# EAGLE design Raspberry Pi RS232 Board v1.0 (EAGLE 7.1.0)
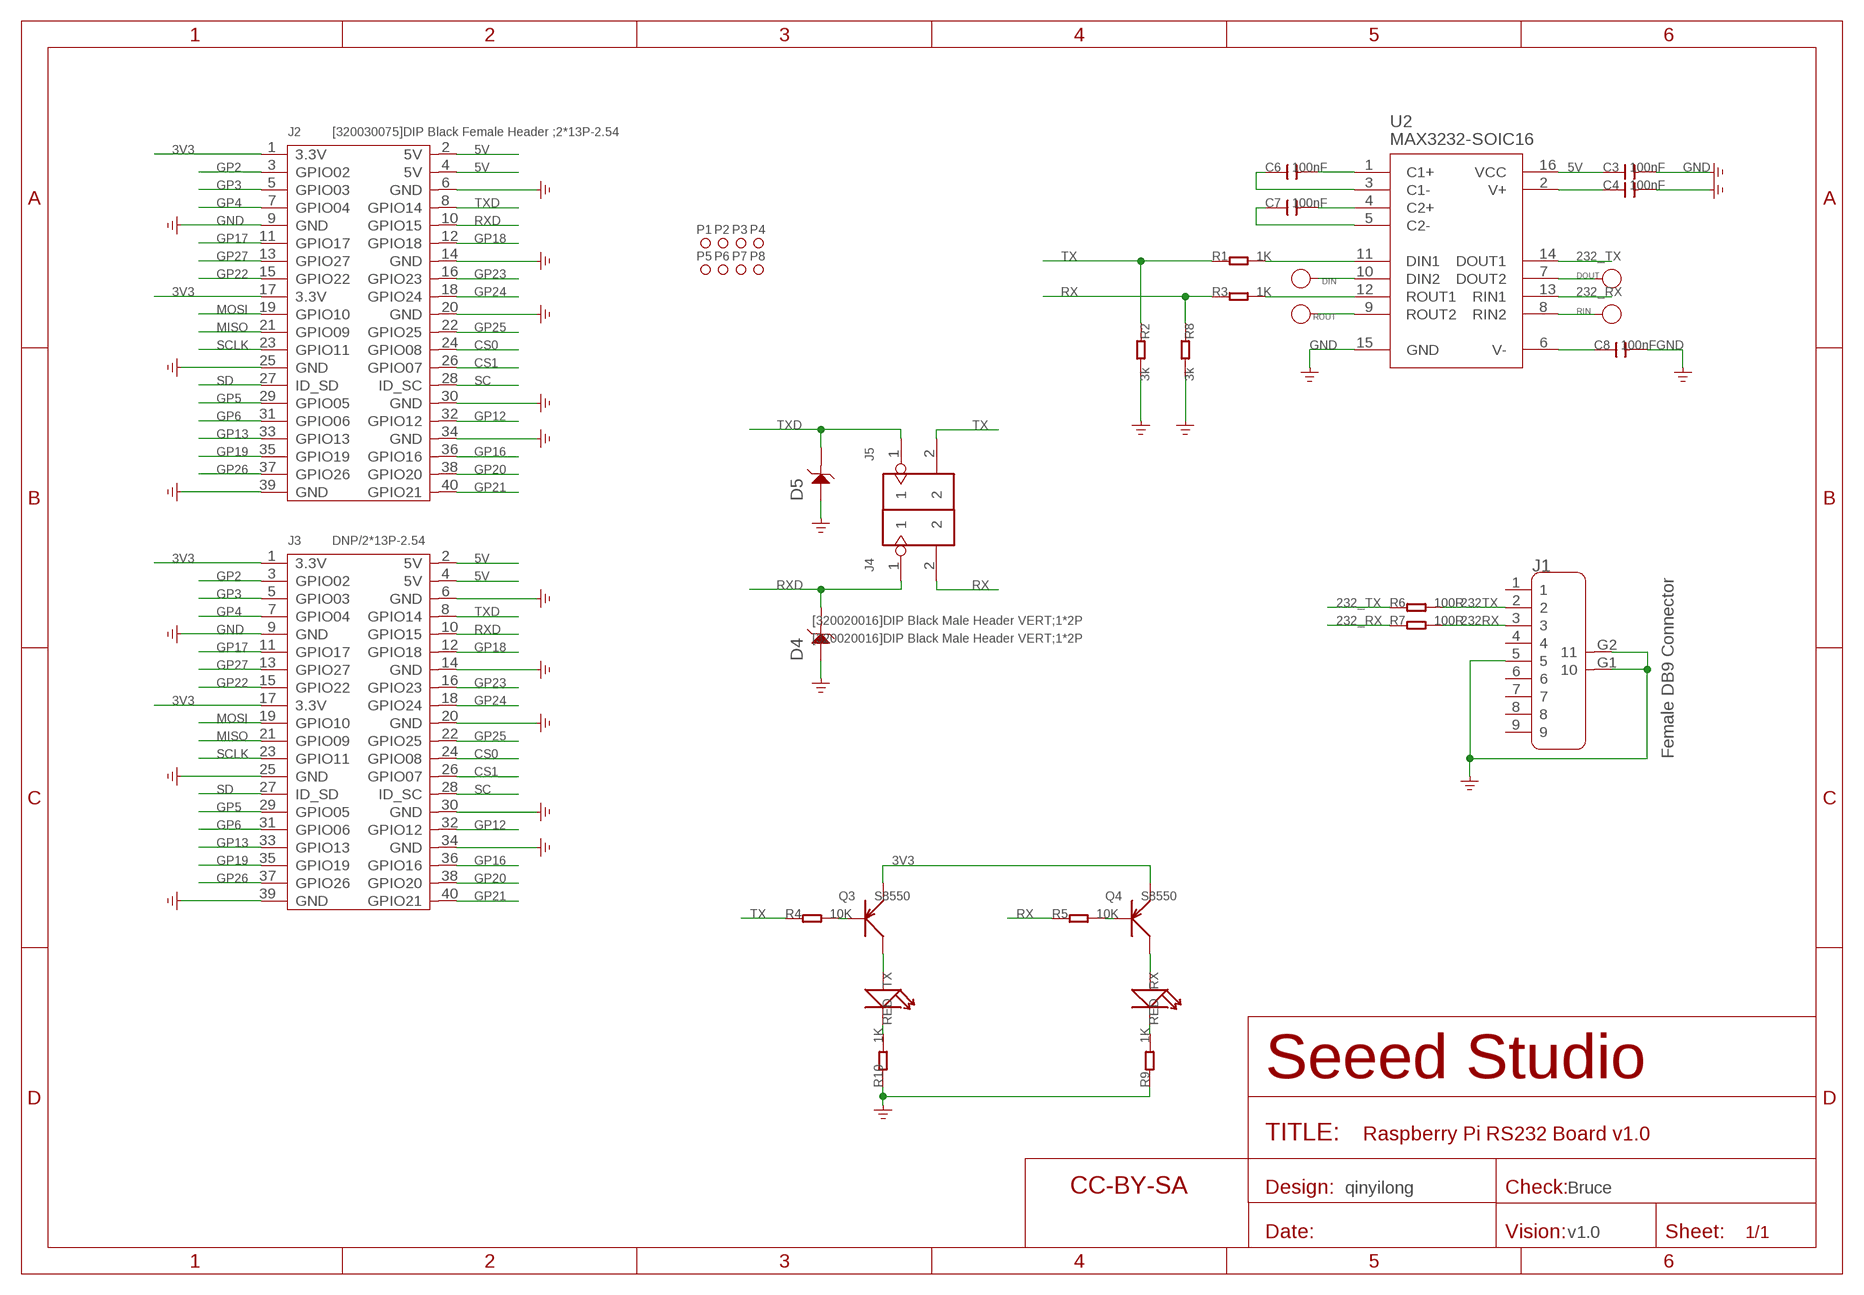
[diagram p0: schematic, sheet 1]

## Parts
C3  100nF  C-0603  [C0603]
C4  100nF  C-0603  [C0603]
C6  100nF  C-0603  [C0603]
C7  100nF  C-0603  [C0603]
C8  100nF  C-0603  [C0603]
D4  DNP  D-ESD-2P'CESD5V0D1'  [SOD123-2.7X1.6]
D5  DNP  D-ESD-2P'CESD5V0D1'  [SOD123-2.7X1.6]
DIN  DNP  PAD-TEST-POINT'4080'  [PAD_4080]
DOUT  DNP  PAD-TEST-POINT'4080'  [PAD_4080]
J1  Female DB9 Connector  DB9'FEMAL'  [DB9]
J2  [320030075]DIP Black Female Header ;2*13P-2.54  HEADER-2X20P  [2X20P-2.54-65/35MIL]
J3  DNP/2*13P-2.54  HEADER-2X20P  [2X20P-2.54-65/35MIL]
J4  [320020016]DIP Black Male Header VERT;1*2P  HEADER-2P-65/35MIL  [2P-2.54-65/35MIL]
J5  [320020016]DIP Black Male Header VERT;1*2P  HEADER-2P-65/35MIL  [2P-2.54-65/35MIL]
P1  PAD-MARK'ANNULAR'  [ROUND-MARK-1.0]
P2  PAD-MARK'ANNULAR'  [ROUND-MARK-1.0]
P3  PAD-MARK'ANNULAR'  [ROUND-MARK-1.0]
P4  PAD-MARK'ANNULAR'  [ROUND-MARK-1.0]
P5  PAD-MARK'ANNULAR'  [ROUND-MARK-1.0]
P6  PAD-MARK'ANNULAR'  [ROUND-MARK-1.0]
P7  PAD-MARK'ANNULAR'  [ROUND-MARK-1.0]
P8  PAD-MARK'ANNULAR'  [ROUND-MARK-1.0]
Q3  S8550  TRANSISTOR-PNP-SOT23  [SOT23]
Q4  S8550  TRANSISTOR-PNP-SOT23  [SOT23]
R1  1K  R-0603  [R0603]
R2  3k  R-0603  [R0603]
R3  1K  R-0603  [R0603]
R4  10K  R-0603  [R0603]
R5  10K  R-0603  [R0603]
R6  100R  R-0603  [R0603]
R7  100R  R-0603  [R0603]
R8  3k  R-0603  [R0603]
R9  1K  R-0603  [R0603]
R10  1K  R-0603  [R0603]
RIN  DNP  PAD-TEST-POINT'4080'  [PAD_4080]
ROUT  DNP  PAD-TEST-POINT'4080'  [PAD_4080]
RX  RED  LED'0603'  [LED-0603]
TX  RED  LED'0603'  [LED-0603]
U2  MAX3232-SOIC16  [SOIC16]
U$2  SEEEDSTUDIO-OPEN-SCH-FRAME  [SEEEDSTUDIO-PCB-FRAME]

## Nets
3V3: J2.1(3.3V) J2.17(3.3V) J3.1(3.3V) J3.17(3.3V) Q3.2(E) Q4.2(E)
5V: C3.1 J2.2(5V) J2.4(5V) J3.2(5V) J3.4(5V) U2.16(VCC)
232_RX: R7.1 U2.13(RIN1)
232_TX: R6.1 U2.14(DOUT1)
232RX: J1.3 R7.2
232TX: J1.2 R6.2
CS0: J2.24(GPIO08) J3.24(GPIO08)
CS1: J2.26(GPIO07) J3.26(GPIO07)
GND: C3.2 C4.2 C8.2 D4.1 D5.1 J1.5 J1.G1 J1.G2 J2.6(GND) J2.9(GND) J2.14(GND) J2.20(GND) J2.25(GND) J2.30(GND) J2.34(GND) J2.39(GND) J3.6(GND) J3.9(GND) J3.14(GND) J3.20(GND) J3.25(GND) J3.30(GND) J3.34(GND) J3.39(GND) R2.2 R8.2 R9.1 R10.1 U2.15(GND) ; supply symbol labelled GND_POWER
GP2: J2.3(GPIO02) J3.3(GPIO02)
GP3: J2.5(GPIO03) J3.5(GPIO03)
GP4: J2.7(GPIO04) J3.7(GPIO04)
GP5: J2.29(GPIO05) J3.29(GPIO05)
GP6: J2.31(GPIO06) J3.31(GPIO06)
GP12: J2.32(GPIO12) J3.32(GPIO12)
GP13: J2.33(GPIO13) J3.33(GPIO13)
GP16: J2.36(GPIO16) J3.36(GPIO16)
GP17: J2.11(GPIO17) J3.11(GPIO17)
GP18: J2.12(GPIO18) J3.12(GPIO18)
GP19: J2.35(GPIO19) J3.35(GPIO19)
GP20: J2.38(GPIO20) J3.38(GPIO20)
GP21: J2.40(GPIO21) J3.40(GPIO21)
GP22: J2.15(GPIO22) J3.15(GPIO22)
GP23: J2.16(GPIO23) J3.16(GPIO23)
GP24: J2.18(GPIO24) J3.18(GPIO24)
GP25: J2.22(GPIO25) J3.22(GPIO25)
GP26: J2.37(GPIO26) J3.37(GPIO26)
GP27: J2.13(GPIO27) J3.13(GPIO27)
MISO: J2.21(GPIO09) J3.21(GPIO09)
MOSI: J2.19(GPIO10) J3.19(GPIO10)
N$1: C6.2 U2.1(C1+)
N$3: C6.1 U2.3(C1-)
N$5: DIN.1(T) U2.10(DIN2)
N$6: ROUT.1(T) U2.9(ROUT2)
N$7: C7.2 U2.4(C2+)
N$8: C7.1 U2.5(C2-)
N$9: C8.1 U2.6(V-)
N$10: C4.1 U2.2(V+)
N$11: Q3.3(C) TX.+
N$14: Q4.3(C) RX.+
N$46: DOUT.1(T) U2.7(DOUT2)
N$47: RIN.1(T) U2.8(RIN2)
N$49: Q3.1(B) R4.2
N$50: Q4.1(B) R5.2
N$51: R10.2 TX.-
N$52: R9.2 RX.-
N$108: R1.2 U2.11(DIN1)
N$189: R3.2 U2.12(ROUT1)
RX: J4.2 R3.1 R5.1 R8.1
RXD: D4.2 J2.10(GPIO15) J3.10(GPIO15) J4.1
SC: J2.28(ID_SC) J3.28(ID_SC)
SCLK: J2.23(GPIO11) J3.23(GPIO11)
SD: J2.27(ID_SD) J3.27(ID_SD)
TX: J5.2 R1.1 R2.1 R4.1
TXD: D5.2 J2.8(GPIO14) J3.8(GPIO14) J5.1
Unconnected: J1.1 J1.4 J1.6 J1.7 J1.8 J1.9

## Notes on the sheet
- qinyilong | Bruce
- v1.0

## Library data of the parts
C3 C4 C6-C8 = Discrete:C*: Ceramic Capacitors
D4 D5 = Discrete:D-ESD-2P: Diodes for Protectiong against ESD
DIN DOUT RIN ROUT = Discrete:PAD-TEST-POINT
J1 = Connector:DB9
J2 J3 = Connector-new:HEADER-2X20P
J4 J5 = Connector-new:HEADER-2P
P1-P8 = Discrete-new:PAD-MARK; PARTNO: DNP
Q3 Q4 = Discrete:TRANSISTOR-PNP*: PNP audion
R1-R10 = Discrete:R*
RX TX = Discrete:LED*
U2 = IC:MAX3232
U$2 = moudle-new:SEEEDSTUDIO-OPEN-SCH-FRAME

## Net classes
0 default: width 0.152 mm, drill 0.305 mm, clearance 0.152 mm

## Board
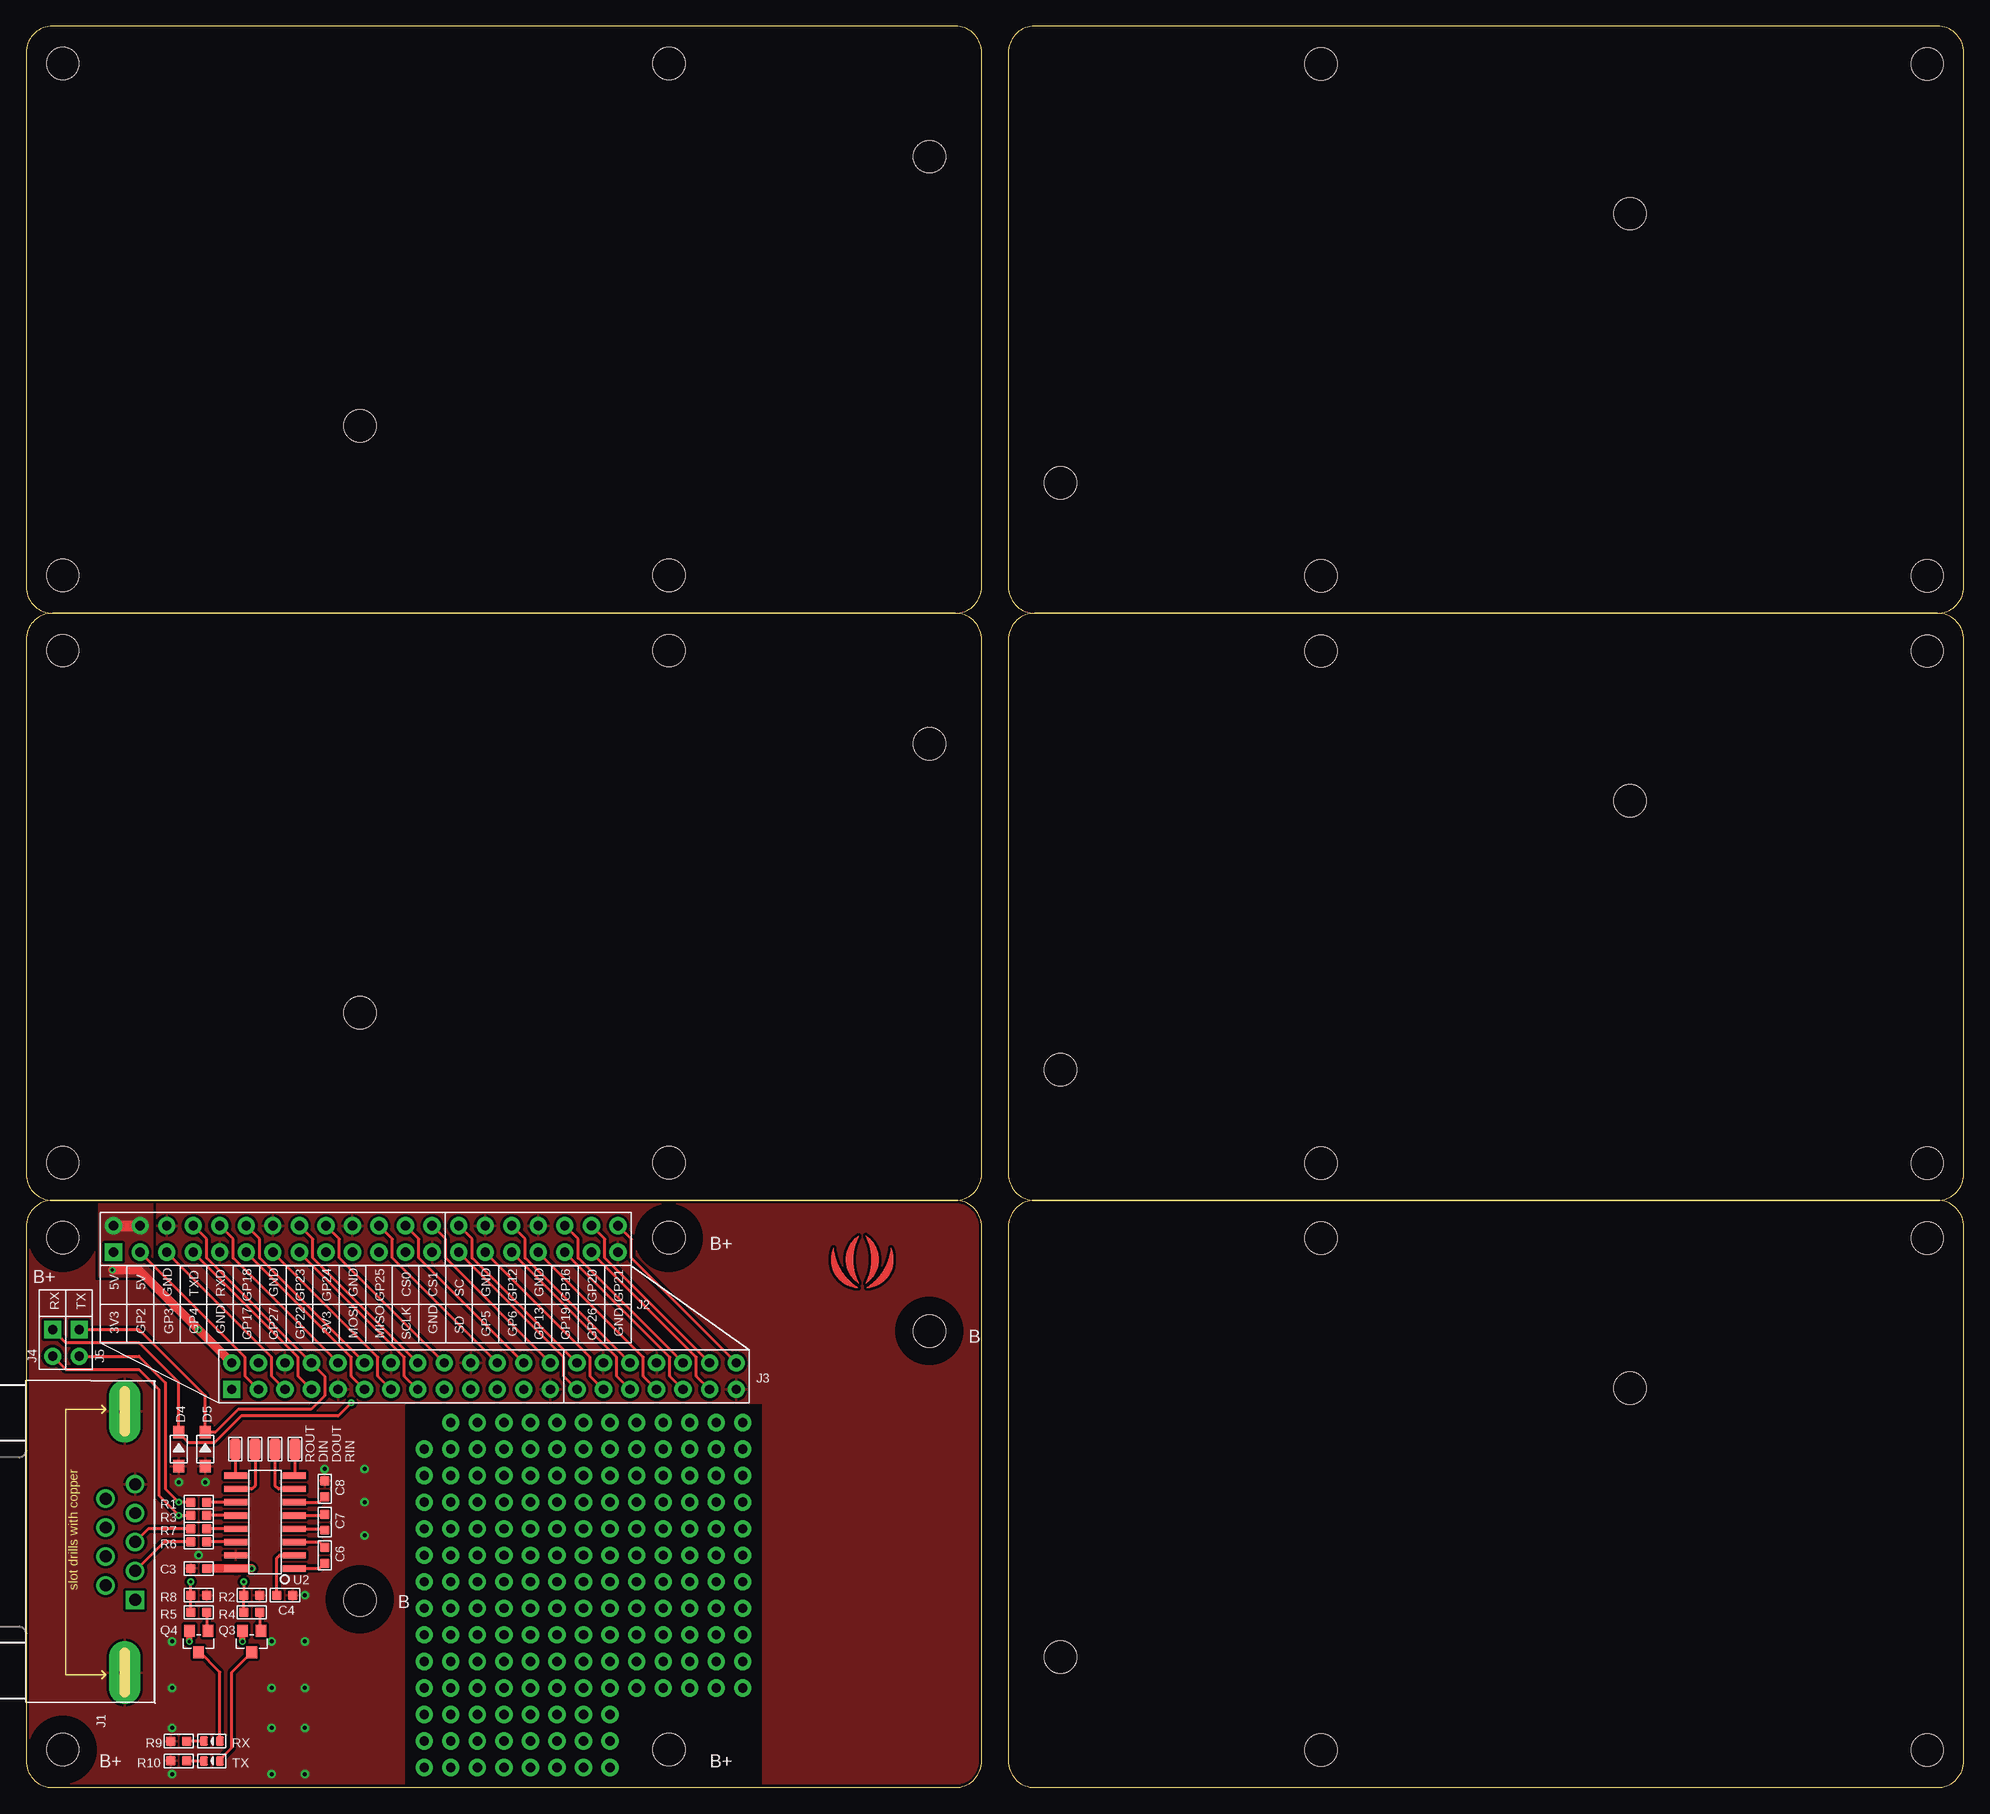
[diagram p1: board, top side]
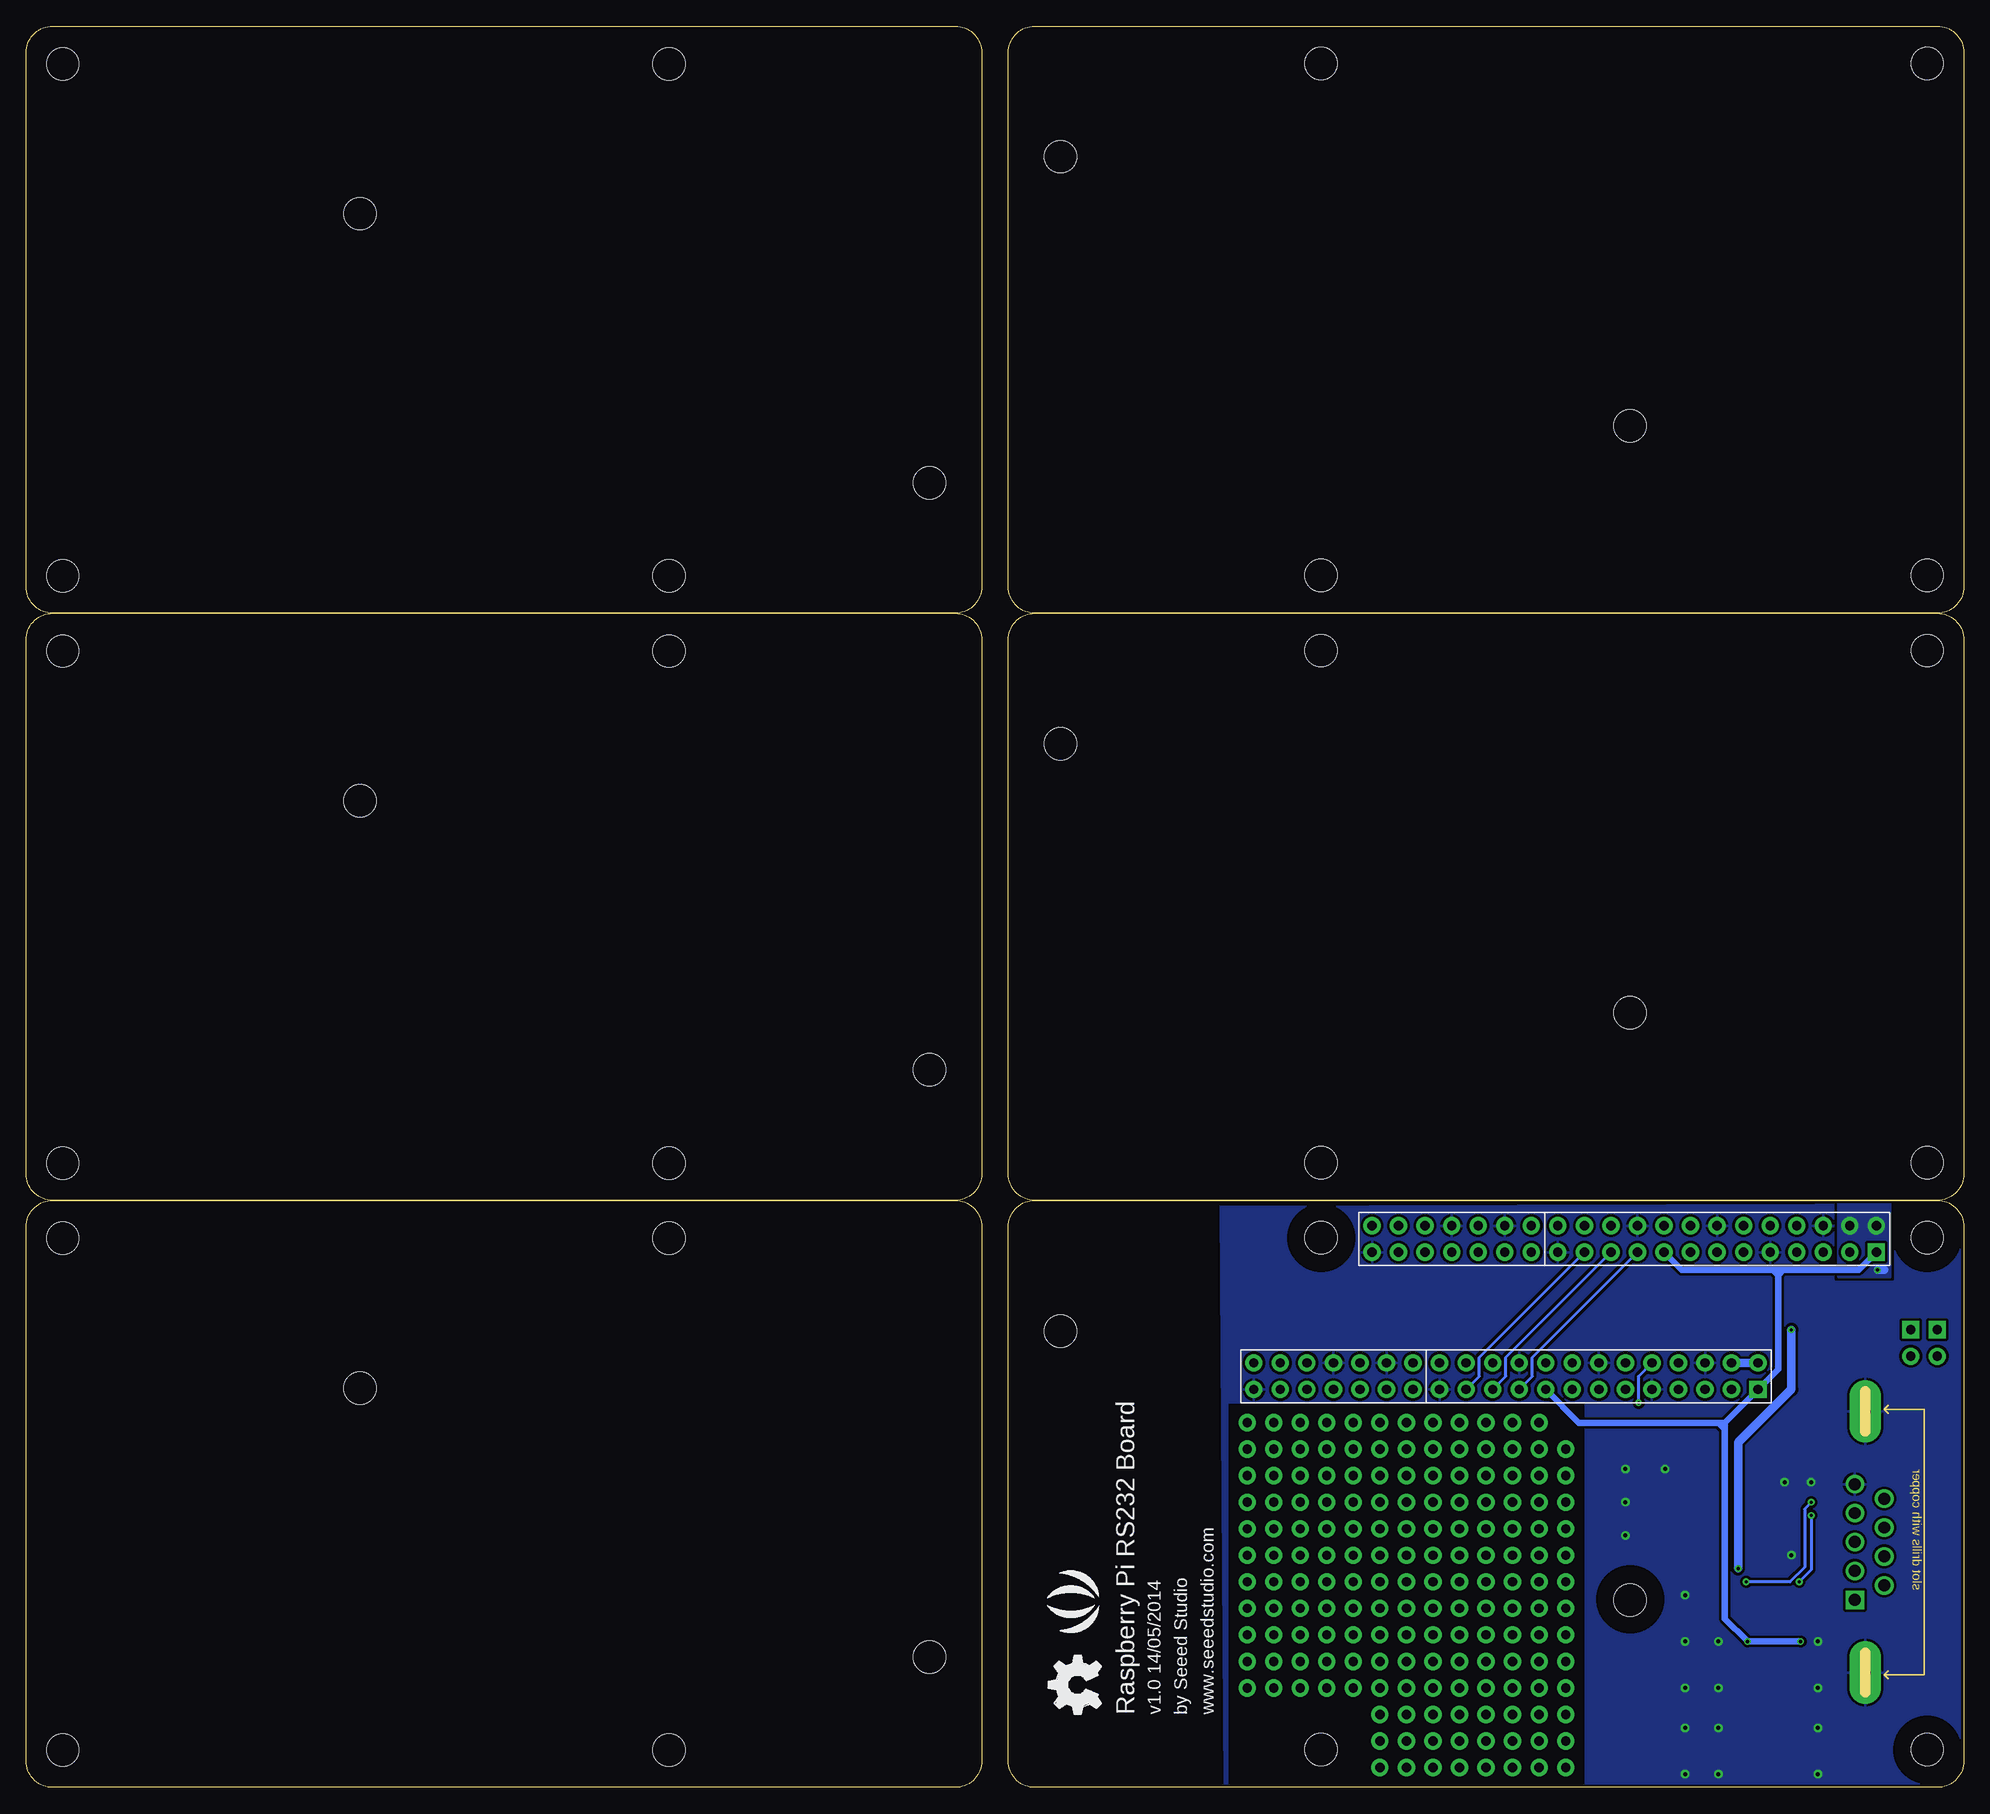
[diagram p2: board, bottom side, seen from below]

Size 185.42 x 168.59 mm. Coordinates in mm from the lower left corner, seen from the top.
Copper layers (1*16): Top 0.035mm / dielectric 1.5mm / Bottom 0.035mm
Design rules "SeeedStudio_2layer_DRU_no_angle_20140221 *": minimum track width 6mil, minimum drill 12mil, track to track 6mil, track to pad 6mil, pad to pad 6mil, via to via 6mil, smd to smd 0mil, copper to edge 10mil, drill to drill 10mil, minimum pad ring 10mil, minimum via ring 6mil, stop-mask expansion 2mil, vias tented up to drill 25mil, thermal gap 10mil
Holes 2.03 mm at 2.54,-5.08 182.88,-5.08 182.88,173.35 2.54,173.35

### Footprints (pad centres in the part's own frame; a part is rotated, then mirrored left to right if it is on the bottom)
C0603 = smd 0.889 x 0.889: 1 -0.762,0; 2 0.762,0
SOD123-2.7X1.6 = smd 1.2 x 1.02: 1 -1.635,0; 2 1.635,0
PAD_4080 = smd 2.032 x 1.016: 1 0,0
DB9 = drill 1.143 pad 1.778 square: 1 5.54,0.9 | drill 1.143 pad 1.778: 2 2.77,0.9; 3 0,0.9; 4 -2.77,0.9; 5 -5.54,0.9; 6 4.155,-1.91; 7 1.385,-1.91; 8 -1.385,-1.91; 9 -4.155,-1.91 | drill 1 pad 3 long: G1 12.5,-0.1; G2 -12.5,-0.1
2X20P-2.54-65/35MIL = drill 0.889 pad 1.651 square: 1 1.27,24.13 | drill 0.889 pad 1.651: 2 -1.27,24.13; 3 1.27,21.59; 4 -1.27,21.59; 5 1.27,19.05; 6 -1.27,19.05; 7 1.27,16.51; 8 -1.27,16.51; 9 1.27,13.97; 10 -1.27,13.97; 11 1.27,11.43; 12 -1.27,11.43; 13 1.27,8.89; 14 -1.27,8.89; 15 1.27,6.35; 16 -1.27,6.35; 17 1.27,3.81; 18 -1.27,3.81; 19 1.27,1.27; 20 -1.27,1.27; 21 1.27,-1.27; 22 -1.27,-1.27; 23 1.27,-3.81; 24 -1.27,-3.81; 25 1.27,-6.35; 26 -1.27,-6.35; 27 1.27,-8.89; 28 -1.27,-8.89; 29 1.27,-11.43; 30 -1.27,-11.43; 31 1.27,-13.97; 32 -1.27,-13.97; 33 1.27,-16.51; 34 -1.27,-16.51; 35 1.27,-19.05; 36 -1.27,-19.05; 37 1.27,-21.59; 38 -1.27,-21.59; 39 1.27,-24.13; 40 -1.27,-24.13
2P-2.54-65/35MIL = drill 0.889 pad 1.651 square: 1 0,1.27 | drill 0.889 pad 1.651: 2 0,-1.27
ROUND-MARK-1.0 = smd 1.016 x 1.016: P$1 0,0
SOT23 = smd 1.016 x 1.143: 1 -0.889,-1.016; 2 0.889,-1.016; 3 0,1.016
R0603 = smd 0.889 x 0.889: 1 -0.762,0; 2 0.762,0
LED-0603 = smd 0.762 x 0.889: + -0.762,0; - 0.762,0
SOIC16 = smd 0.6 x 2.2: 1 -4.445,-2.8; 2 -3.175,-2.8; 3 -1.905,-2.8; 4 -0.635,-2.8; 5 0.635,-2.8; 6 1.905,-2.8; 7 3.175,-2.8; 8 4.445,-2.8; 9 4.445,2.8; 10 3.175,2.8; 11 1.905,2.8; 12 0.635,2.8; 13 -0.635,2.8; 14 -1.905,2.8; 15 -3.175,2.8; 16 -4.445,2.8
RASPBERRY-PI-B+/B = hole 3.1: 3.503,52.622; 3.503,3.622; 61.503,52.622; 61.503,3.622; 31.951,17.951; 86.431,43.7

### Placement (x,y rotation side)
C3  16.51,20.95 180 top
C4  24.77,18.41 0 top
C6  28.57,22.23 270 top
C7  28.57,25.4 270 top
C8  28.57,28.57 90 top
D4  14.61,32.38 90 top
D5  17.14,32.38 90 top
DIN  21.91,32.38 90 top
DOUT  23.81,32.38 90 top
J1  9.53,23.5 270 top
J2  32.5,52.5 270 bottom
J3  43.81,39.37 270 bottom
J4  2.54,42.55 0 top
J5  5.08,42.55 0 top
P1  not placed on the board
P2  not placed on the board
P3  not placed on the board
P4  not placed on the board
P5  not placed on the board
P6  not placed on the board
P7  not placed on the board
P8  not placed on the board
Q3  21.59,13.97 180 top
Q4  16.51,13.97 180 top
R1  16.51,27.3 0 top
R2  21.59,18.41 0 top
R3  16.51,26.04 0 top
R4  21.59,16.76 0 top
R5  16.51,16.76 0 top
R6  16.51,23.5 180 top
R7  16.51,24.77 180 top
R8  16.51,18.41 0 top
R9  14.61,4.45 0 top
R10  14.61,2.54 0 top
RIN  25.72,32.38 90 top
ROUT  20,32.38 270 top
RX  17.78,4.45 180 top
TX  17.78,2.54 180 top
U2  22.86,25.4 90 top
U$2  not placed on the board
U$12  [OSHW_FILLX200_NOTEXT]  82.55,6.99 90 bottom
U$17  [SEEED-SILK-280*268MIL]  84.45,17.78 90 bottom
U$29  [RASPBERRY-PI-B+/B]  0,0 0 top
U$30  [SEEED-COPPER-280*268MIL]  80.01,49.53 0 top
U$31  [RASPBERRY-PI-B+/B]  0,56.2 0 top
U$32  [RASPBERRY-PI-B+/B]  0,112.39 0 top
U$33  [RASPBERRY-PI-B+/B]  185.42,56.2 180 top
U$34  [RASPBERRY-PI-B+/B]  185.42,112.39 180 top
U$35  [RASPBERRY-PI-B+/B]  185.42,168.59 180 top

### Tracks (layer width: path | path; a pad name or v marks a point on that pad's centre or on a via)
3V3  (via drill 0.3 pad 0.64)
  Top 0.61: Q4.2 v15.62,13.97 | v20.7,13.97 Q3.2
  Bottom 0.61: v15.62,13.97 v20.7,13.97 22.86,16.13 22.86,34.16 22.86,34.29 | 22.86,34.92 J3.1 17.78,40.01 17.78,49.02 | J3.17 36.83,34.92 23.5,34.92 | 17.78,49.02 17.78,49.53 | 17.78,49.53 17.27,49.53 | 17.27,49.53 10.07,49.53 J2.1 | 17.78,49.53 18.29,49.53 | 18.29,49.53 26.99,49.53 J2.17 | 22.86,34.29 22.86,34.92 | 17.27,49.53 17.78,49.02 | 17.78,49.02 18.29,49.53 | 22.86,34.92 23.5,34.92 | 22.86,34.29 23.5,34.92
5V  (via drill 0.3 pad 0.64)
  Top 0.813: v21.59,20.95 U2.16 C3.1 | v8.26,49.53 10.79,49.53 v16.51,43.81 J3.2
  Top 1.016: J2.4 J2.2
  Bottom 0.813: J3.4 J3.2 | v8.26,49.53 7.62,49.53 | v21.59,20.95 21.59,33.02 16.51,38.1 v16.51,43.81
  pour Top (isolate 0.254, no thermals): 6.99,56.01 12.06,56.01 12.06,48.9 6.99,48.9
  pour Bottom (isolate 0.254, no thermals): 6.99,56.01 12.06,56.01 12.06,48.9 6.99,48.9
232_RX
  Top 0.305: U2.13 R7.1
232_TX
  Top 0.305: U2.14 R6.1
232RX
  Top 0.305: R7.2 11.7,24.77 J1.3
232TX
  Top 0.305: R6.2 13.2,23.5 J1.2
CS0
  Top 0.305: J3.24 37.59,50.67 37.59,52.49 J2.24
CS1
  Top 0.305: J3.26 40.13,50.67 40.13,52.49 J2.26
GND  (via drill 0.38 pad 0.81)
  other vias: 16.51,22.23 14.61,29.21 17.14,29.21 28.57,30.48 26.67,18.41 26.67,13.97 32.38,30.48 32.38,27.3 32.38,24.13 13.97,5.71 13.97,1.27 13.97,9.53 13.97,13.97 23.5,13.97 23.5,9.53 23.5,5.71 23.5,1.27 26.67,9.53 26.67,5.71 26.67,1.27
  pour Top (isolate 0.254, rank 6): 0,0 36.2,0 36.2,36.83 70.48,36.83 70.48,0 91.44,0 91.44,55.88 0,55.88 0,0.13
  pour Bottom (isolate 0.254, rank 6): 0,0 36.2,0 36.2,36.83 70.48,36.83 70.48,0 70.74,0 71.12,55.63 0,55.88
GP2
  Top 0.305: J3.3 20.95,39.37 20.95,41.19 J2.3
GP3
  Top 0.305: J3.5 23.5,39.37 23.5,41.19 J2.5
GP4
  Top 0.305: J3.7 26.04,39.37 26.04,41.19 J2.7
GP5
  Top 0.305: J3.29 53.98,39.37 53.98,41.19 J2.29
GP6
  Top 0.305: J3.31 56.52,39.37 56.52,41.19 J2.31
GP12
  Top 0.305: J3.32 47.75,50.67 47.75,52.49 J2.32
GP13
  Top 0.305: J3.33 59.05,39.37 59.05,41.19 J2.33
GP16
  Top 0.305: J3.36 52.83,50.67 52.83,52.49 J2.36
GP17
  Top 0.305: J3.11 31.11,39.37 31.11,41.19 J2.11
GP18
  Top 0.305: J3.12 22.35,50.67 22.35,52.49 J2.12
GP19
  Top 0.305: J3.35 61.59,39.37 61.59,41.19 J2.35
GP20
  Top 0.305: J3.38 55.37,50.67 55.37,52.49 J2.38
GP21
  Top 0.305: J3.40 57.91,50.67 57.91,52.49 J2.40
GP22
  Top 0.305: J3.15 36.2,39.37 36.2,41.19 J2.15
GP23
  Top 0.305: J3.16 27.43,50.67 27.43,52.49 J2.16
GP24
  Top 0.305: J3.18 29.97,50.67 29.97,52.49 J2.18
GP25
  Top 0.305: J3.22 35.05,50.67 35.05,52.49 J2.22
GP26
  Top 0.305: J3.37 64.14,39.37 64.14,41.19 J2.37
GP27
  Top 0.305: J3.13 33.66,39.37 33.66,41.19 J2.13
MISO
  Bottom 0.305: J3.21 43.81,39.37 43.81,41.19 J2.21
MOSI
  Bottom 0.305: J3.19 41.27,39.37 41.27,41.19 J2.19
N$1
  Top 0.305: U2.1 28.07,20.95 C6.2
N$2  (via drill 0.89 pad 1.65)
  other vias: 38.1,32.38
N$3
  Top 0.305: U2.3 28.07,23.5 C6.1
N$4  (via drill 0.89 pad 1.65)
  other vias: 40.64,32.38
N$5
  Top 0.305: DIN.1 21.91,28.89 21.59,28.57 U2.10
N$6
  Top 0.305: ROUT.1 20,29.9 U2.9
N$7
  Top 0.305: U2.4 28.45,24.77 C7.2
N$8
  Top 0.305: U2.5 28.45,26.04 C7.1
N$9
  Top 0.305: U2.6 28.07,27.3 C8.1
N$10
  Top 0.305: C4.1 24,21.97 24.26,22.23 U2.2
N$11
  Top 0.305: TX.+ 18.54,2.67 19.68,3.81 19.68,11.05 Q3.3
N$12  (via drill 0.89 pad 1.65)
  other vias: 38.1,24.77
N$13  (via drill 0.89 pad 1.65)
  other vias: 38.1,22.23
N$14
  Top 0.305: RX.+ 18.54,11.05 16.51,13.08 Q4.3
N$15  (via drill 0.89 pad 1.65)
  other vias: 38.1,19.68
N$16  (via drill 0.89 pad 1.65)
  other vias: 40.64,24.77
N$17  (via drill 0.89 pad 1.65)
  other vias: 40.64,22.23
N$18  (via drill 0.89 pad 1.65)
  other vias: 40.64,19.68
N$19  (via drill 0.89 pad 1.65)
  other vias: 43.18,24.77
N$20  (via drill 0.89 pad 1.65)
  other vias: 43.18,22.23
N$21  (via drill 0.89 pad 1.65)
  other vias: 43.18,19.68
N$22  (via drill 0.89 pad 1.65)
  other vias: 45.72,24.77
N$23  (via drill 0.89 pad 1.65)
  other vias: 45.72,22.23
N$24  (via drill 0.89 pad 1.65)
  other vias: 45.72,19.68
N$25  (via drill 0.89 pad 1.65)
  other vias: 48.26,24.77
N$26  (via drill 0.89 pad 1.65)
  other vias: 48.26,22.23
N$27  (via drill 0.89 pad 1.65)
  other vias: 48.26,19.68
N$28  (via drill 0.89 pad 1.65)
  other vias: 50.8,24.77
N$29  (via drill 0.89 pad 1.65)
  other vias: 50.8,22.23
N$30  (via drill 0.89 pad 1.65)
  other vias: 50.8,19.68
N$31  (via drill 0.89 pad 1.65)
  other vias: 53.34,24.77
N$32  (via drill 0.89 pad 1.65)
  other vias: 53.34,22.23
N$33  (via drill 0.89 pad 1.65)
  other vias: 53.34,19.68
N$34  (via drill 0.89 pad 1.65)
  other vias: 55.88,24.77
N$35  (via drill 0.89 pad 1.65)
  other vias: 55.88,22.23
N$36  (via drill 0.89 pad 1.65)
  other vias: 55.88,19.68
N$37  (via drill 0.89 pad 1.65)
  other vias: 58.42,24.77
N$38  (via drill 0.89 pad 1.65)
  other vias: 58.42,22.23
N$39  (via drill 0.89 pad 1.65)
  other vias: 58.42,19.68
N$40  (via drill 0.89 pad 1.65)
  other vias: 60.96,24.77
N$41  (via drill 0.89 pad 1.65)
  other vias: 60.96,22.23
N$42  (via drill 0.89 pad 1.65)
  other vias: 60.96,19.68
N$43  (via drill 0.89 pad 1.65)
  other vias: 43.18,32.38
N$44  (via drill 0.89 pad 1.65)
  other vias: 45.72,32.38
N$45  (via drill 0.89 pad 1.65)
  other vias: 48.26,32.38
N$46
  Top 0.305: DOUT.1 23.81,28.89 24.07,28.64 24.13,28.57 U2.7
N$47
  Top 0.305: RIN.1 25.72,29.9 U2.8
N$48  (via drill 0.89 pad 1.65)
  other vias: 50.8,32.38
N$49
  Top 0.305: R4.2 22.35,15.11 Q3.1
N$50
  Top 0.305: R5.2 17.27,15.11 Q4.1
N$51
  Top 0.305: R10.2 TX.-
N$52
  Top 0.305: RX.- R9.2
N$53  (via drill 0.89 pad 1.65)
  other vias: 53.34,32.38
N$54  (via drill 0.89 pad 1.65)
  other vias: 38.1,17.14
N$55  (via drill 0.89 pad 1.65)
  other vias: 38.1,27.3
N$56  (via drill 0.89 pad 1.65)
  other vias: 38.1,14.61
N$57  (via drill 0.89 pad 1.65)
  other vias: 38.1,12.06
N$58  (via drill 0.89 pad 1.65)
  other vias: 40.64,17.14
N$59  (via drill 0.89 pad 1.65)
  other vias: 40.64,14.61
N$60  (via drill 0.89 pad 1.65)
  other vias: 40.64,12.06
N$61  (via drill 0.89 pad 1.65)
  other vias: 43.18,17.14
N$62  (via drill 0.89 pad 1.65)
  other vias: 43.18,14.61
N$63  (via drill 0.89 pad 1.65)
  other vias: 43.18,12.06
N$64  (via drill 0.89 pad 1.65)
  other vias: 45.72,17.14
N$65  (via drill 0.89 pad 1.65)
  other vias: 45.72,14.61
N$66  (via drill 0.89 pad 1.65)
  other vias: 45.72,12.06
N$67  (via drill 0.89 pad 1.65)
  other vias: 48.26,17.14
N$68  (via drill 0.89 pad 1.65)
  other vias: 48.26,14.61
N$69  (via drill 0.89 pad 1.65)
  other vias: 48.26,12.06
N$70  (via drill 0.89 pad 1.65)
  other vias: 50.8,17.14
N$71  (via drill 0.89 pad 1.65)
  other vias: 50.8,14.61
N$72  (via drill 0.89 pad 1.65)
  other vias: 50.8,12.06
N$73  (via drill 0.89 pad 1.65)
  other vias: 53.34,17.14
N$74  (via drill 0.89 pad 1.65)
  other vias: 53.34,14.61
N$75  (via drill 0.89 pad 1.65)
  other vias: 53.34,12.06
N$76  (via drill 0.89 pad 1.65)
  other vias: 55.88,17.14
N$77  (via drill 0.89 pad 1.65)
  other vias: 55.88,14.61
N$78  (via drill 0.89 pad 1.65)
  other vias: 55.88,12.06
N$79  (via drill 0.89 pad 1.65)
  other vias: 58.42,17.14
N$80  (via drill 0.89 pad 1.65)
  other vias: 58.42,14.61
N$81  (via drill 0.89 pad 1.65)
  other vias: 58.42,12.06
N$82  (via drill 0.89 pad 1.65)
  other vias: 60.96,17.14
N$83  (via drill 0.89 pad 1.65)
  other vias: 60.96,14.61
N$84  (via drill 0.89 pad 1.65)
  other vias: 60.96,12.06
N$85  (via drill 0.89 pad 1.65)
  other vias: 55.88,32.38
N$86  (via drill 0.89 pad 1.65)
  other vias: 58.42,32.38
N$87  (via drill 0.89 pad 1.65)
  other vias: 60.96,32.38
N$88  (via drill 0.89 pad 1.65)
  other vias: 38.1,6.99
N$89  (via drill 0.89 pad 1.65)
  other vias: 40.64,6.99
N$90  (via drill 0.89 pad 1.65)
  other vias: 43.18,6.99
N$91  (via drill 0.89 pad 1.65)
  other vias: 45.72,6.99
N$92  (via drill 0.89 pad 1.65)
  other vias: 48.26,6.99
N$93  (via drill 0.89 pad 1.65)
  other vias: 50.8,6.99
N$94  (via drill 0.89 pad 1.65)
  other vias: 38.1,9.53
N$95  (via drill 0.89 pad 1.65)
  other vias: 53.34,6.99
N$96  (via drill 0.89 pad 1.65)
  other vias: 55.88,6.99
N$97  (via drill 0.89 pad 1.65)
  other vias: 38.1,4.45
N$98  (via drill 0.89 pad 1.65)
  other vias: 40.64,4.45
N$99  (via drill 0.89 pad 1.65)
  other vias: 40.64,27.3
N$100  (via drill 0.89 pad 1.65)
  other vias: 40.64,9.53
N$101  (via drill 0.89 pad 1.65)
  other vias: 43.18,4.45
N$102  (via drill 0.89 pad 1.65)
  other vias: 45.72,4.45
N$103  (via drill 0.89 pad 1.65)
  other vias: 48.26,4.45
N$104  (via drill 0.89 pad 1.65)
  other vias: 50.8,4.45
N$105  (via drill 0.89 pad 1.65)
  other vias: 53.34,4.45
N$106  (via drill 0.89 pad 1.65)
  other vias: 45.72,9.53
N$107  (via drill 0.89 pad 1.65)
  other vias: 55.88,4.45
N$108
  Top 0.305: U2.11 R1.2 17.14,27.3
N$109  (via drill 0.89 pad 1.65)
  other vias: 48.26,9.53
N$110  (via drill 0.89 pad 1.65)
  other vias: 40.64,34.92
N$111  (via drill 0.89 pad 1.65)
  other vias: 43.18,34.92
N$112  (via drill 0.89 pad 1.65)
  other vias: 50.8,9.53
N$113  (via drill 0.89 pad 1.65)
  other vias: 45.72,34.92
N$114  (via drill 0.89 pad 1.65)
  other vias: 48.26,34.92
N$115  (via drill 0.89 pad 1.65)
  other vias: 53.34,9.53
N$116  (via drill 0.89 pad 1.65)
  other vias: 50.8,34.92
N$117  (via drill 0.89 pad 1.65)
  other vias: 53.34,34.92
N$118  (via drill 0.89 pad 1.65)
  other vias: 55.88,9.53
N$119  (via drill 0.89 pad 1.65)
  other vias: 55.88,34.92
N$120  (via drill 0.89 pad 1.65)
  other vias: 58.42,34.92
N$121  (via drill 0.89 pad 1.65)
  other vias: 58.42,9.53
N$122  (via drill 0.89 pad 1.65)
  other vias: 60.96,34.92
N$124  (via drill 0.89 pad 1.65)
  other vias: 60.96,9.53
N$125  (via drill 0.89 pad 1.65)
  other vias: 38.1,1.91
N$126  (via drill 0.89 pad 1.65)
  other vias: 40.64,1.91
N$127  (via drill 0.89 pad 1.65)
  other vias: 43.18,1.91
N$128  (via drill 0.89 pad 1.65)
  other vias: 45.72,1.91
N$129  (via drill 0.89 pad 1.65)
  other vias: 48.26,1.91
N$130  (via drill 0.89 pad 1.65)
  other vias: 50.8,1.91
N$131  (via drill 0.89 pad 1.65)
  other vias: 53.34,1.91
N$132  (via drill 0.89 pad 1.65)
  other vias: 55.88,1.91
N$133  (via drill 0.89 pad 1.65)
  other vias: 63.5,34.92
N$134  (via drill 0.89 pad 1.65)
  other vias: 63.5,32.38
N$135  (via drill 0.89 pad 1.65)
  other vias: 63.5,29.84
N$136  (via drill 0.89 pad 1.65)
  other vias: 63.5,27.3
N$137  (via drill 0.89 pad 1.65)
  other vias: 63.5,24.77
N$138  (via drill 0.89 pad 1.65)
  other vias: 63.5,22.23
N$139  (via drill 0.89 pad 1.65)
  other vias: 63.5,19.68
N$141  (via drill 0.89 pad 1.65)
  other vias: 63.5,17.14
N$142  (via drill 0.89 pad 1.65)
  other vias: 63.5,14.61
N$143  (via drill 0.89 pad 1.65)
  other vias: 43.18,27.3
N$144  (via drill 0.89 pad 1.65)
  other vias: 63.5,12.06
N$145  (via drill 0.89 pad 1.65)
  other vias: 63.5,9.53
N$146  (via drill 0.89 pad 1.65)
  other vias: 66.04,27.3
N$147  (via drill 0.89 pad 1.65)
  other vias: 66.04,24.77
N$148  (via drill 0.89 pad 1.65)
  other vias: 66.04,22.23
N$156  (via drill 0.89 pad 1.65)
  other vias: 38.1,29.84
N$157  (via drill 0.89 pad 1.65)
  other vias: 40.64,29.84
N$158  (via drill 0.89 pad 1.65)
  other vias: 43.18,29.84
N$159  (via drill 0.89 pad 1.65)
  other vias: 45.72,29.84
N$160  (via drill 0.89 pad 1.65)
  other vias: 48.26,29.84
N$161  (via drill 0.89 pad 1.65)
  other vias: 50.8,29.84
N$162  (via drill 0.89 pad 1.65)
  other vias: 53.34,29.84
N$163  (via drill 0.89 pad 1.65)
  other vias: 55.88,29.84
N$164  (via drill 0.89 pad 1.65)
  other vias: 58.42,29.84
N$165  (via drill 0.89 pad 1.65)
  other vias: 60.96,29.84
N$166  (via drill 0.89 pad 1.65)
  other vias: 66.04,19.68
N$167  (via drill 0.89 pad 1.65)
  other vias: 66.04,17.14
N$168  (via drill 0.89 pad 1.65)
  other vias: 66.04,14.61
N$169  (via drill 0.89 pad 1.65)
  other vias: 66.04,12.06
N$170  (via drill 0.89 pad 1.65)
  other vias: 66.04,9.53
N$171  (via drill 0.89 pad 1.65)
  other vias: 66.04,29.84
N$172  (via drill 0.89 pad 1.65)
  other vias: 66.04,32.38
N$173  (via drill 0.89 pad 1.65)
  other vias: 66.04,34.92
N$174  (via drill 0.89 pad 1.65)
  other vias: 68.58,34.92
N$175  (via drill 0.89 pad 1.65)
  other vias: 68.58,32.38
N$176  (via drill 0.89 pad 1.65)
  other vias: 68.58,29.84
N$177  (via drill 0.89 pad 1.65)
  other vias: 68.58,27.3
N$178  (via drill 0.89 pad 1.65)
  other vias: 68.58,24.77
N$179  (via drill 0.89 pad 1.65)
  other vias: 68.58,22.23
N$180  (via drill 0.89 pad 1.65)
  other vias: 68.58,19.68
N$181  (via drill 0.89 pad 1.65)
  other vias: 68.58,17.14
N$182  (via drill 0.89 pad 1.65)
  other vias: 43.18,9.53
N$185  (via drill 0.89 pad 1.65)
  other vias: 68.58,14.61
N$186  (via drill 0.89 pad 1.65)
  other vias: 68.58,12.06
N$187  (via drill 0.89 pad 1.65)
  other vias: 45.72,27.3
N$188  (via drill 0.89 pad 1.65)
  other vias: 68.58,9.53
N$189
  Top 0.305: U2.12 R3.2
N$231  (via drill 0.89 pad 1.65)
  other vias: 48.26,27.3
N$275  (via drill 0.89 pad 1.65)
  other vias: 50.8,27.3
N$319  (via drill 0.89 pad 1.65)
  other vias: 53.34,27.3
N$363  (via drill 0.89 pad 1.65)
  other vias: 55.88,27.3
N$407  (via drill 0.89 pad 1.65)
  other vias: 58.42,27.3
N$451  (via drill 0.89 pad 1.65)
  other vias: 60.96,27.3
RX  (via drill 0.3 pad 0.64)
  Top 0.305: R5.1 R8.1 15.75,19.56 v15.75,19.68 | J4.2 3.81,40.01 10.79,40.01 12.7,38.1 12.7,27.94 v14.61,26.04 R3.1
  Bottom 0.305: v14.61,26.04 14.61,20.83 v15.75,19.68
RXD  (via drill 0.3 pad 0.64)
  Top 0.305: J4.1 3.81,42.55 10.82,42.55 14.61,38.76 D4.2 14.61,33.91 15.49,33.02 18.03,33.02 20.57,35.56 29.84,35.56 v31.11,36.83 | J3.10 19.81,50.67 19.81,52.49 J2.10
  Bottom 0.305: v31.11,36.83 31.11,39.37 J3.10
SC
  Top 0.305: J3.28 42.67,50.67 42.67,52.49 J2.28
SCLK
  Bottom 0.305: J3.23 46.35,39.37 46.35,41.19 J2.23
SD
  Top 0.305: J3.27 51.44,39.37 51.44,41.19 J2.27
TX  (via drill 0.3 pad 0.64)
  Top 0.305: R4.1 R2.1 v20.83,19.68 | J5.2 10.79,41.27 13.34,38.73 13.34,28.57 v14.61,27.3 R1.1
  Bottom 0.305: v14.61,27.3 15.24,26.67 15.24,21.08 16.64,19.68 v20.83,19.68
TXD
  Top 0.305: J5.1 10.82,43.81 17.14,37.49 D5.2 18.14,34.02 20.32,36.2 27.27,36.2 28.57,37.5 28.57,39.37 J3.8 17.27,50.67 17.27,52.49 J2.8

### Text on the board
tPlace: B+ | B+ | 5V | 5V | GND | TXD | RXD | GP18 | GND | GP23 | GP24 | GND | GP25 | CS0 | CS1 | SC | GND | GP12 | GND | GP16 | RX | TX | GP20 | GP21 | 3V3 | GP2 | GP3 | GP4 | GND | GP17 | GP27 | GP22 | 3V3 | MOSI | MISO | SCLK | GND | SD | GP5 | GP6 | GP13 | GP19 | GP26 | GND | B | B | B+ | B+
bPlace: www.seeedstudio.com | by Seeed Studio | v1.0 14/05/2014 | Raspberry Pi RS232 Board

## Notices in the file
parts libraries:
moudle-new: This work is licensed under the Creative Commons Attribution 4.0 International License.
To view a copy of this license,visit:
http://creativecommons.org/licenses/by-sa/4.0
moudle-new: CC-BY-SA
